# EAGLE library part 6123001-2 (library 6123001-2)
Board to Board & Mezzanine Connectors 0.8FH P08H.5 060 30/Sn TR SC Source: Datasheet
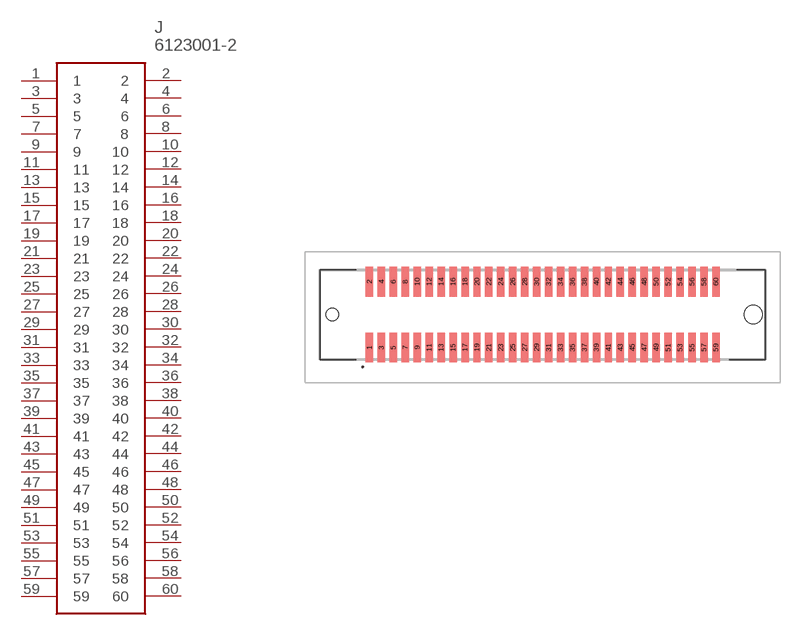
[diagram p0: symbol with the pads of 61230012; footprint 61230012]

Designator prefix J

## 6123001-2 (Arrow_Part_Number: 6123001-2; Arrow_Price-Stock: https://www.arrow.com/en/products/6123001-2/te-connectivity; Description: Board to Board & Mezzanine Connectors 0.8FH P08H.5 060 30/Sn TR SC; Height: 7.8mm; Manufacturer_Name: TE Connectivity; Manufacturer_Part_Number: 6123001-2; Mouser_Part_Number: 571-6123001-2; Mouser_Price-Stock: https://www.mouser.com/Search/Refine.aspx?Keyword=571-6123001-2)  [61230012]
1  1
2  2
3  3
4  4
5  5
6  6
7  7
8  8
9  9
10  10
11  11
12  12
13  13
14  14
15  15
16  16
17  17
18  18
19  19
20  20
21  21
22  22
23  23
24  24
25  25
26  26
27  27
28  28
29  29
30  30
31  31
32  32
33  33
34  34
35  35
36  36
37  37
38  38
39  39
40  40
41  41
42  42
43  43
44  44
45  45
46  46
47  47
48  48
49  49
50  50
51  51
52  52
53  53
54  54
55  55
56  56
57  57
58  58
59  59
60  60

## Footprint 61230012 (pad centres in mm)
6123001-2-2
smd 0.5 x 2: 1 -11.6,-2.2; 2 -11.6,2.2; 3 -10.8,-2.2; 4 -10.8,2.2; 5 -10,-2.2; 6 -10,2.2; 7 -9.2,-2.2; 8 -9.2,2.2; 9 -8.4,-2.2; 10 -8.4,2.2; 11 -7.6,-2.2; 12 -7.6,2.2; 13 -6.8,-2.2; 14 -6.8,2.2; 15 -6,-2.2; 16 -6,2.2; 17 -5.2,-2.2; 18 -5.2,2.2; 19 -4.4,-2.2; 20 -4.4,2.2; 21 -3.6,-2.2; 22 -3.6,2.2; 23 -2.8,-2.2; 24 -2.8,2.2; 25 -2,-2.2; 26 -2,2.2; 27 -1.2,-2.2; 28 -1.2,2.2; 29 -0.4,-2.2; 30 -0.4,2.2; 31 0.4,-2.2; 32 0.4,2.2; 33 1.2,-2.2; 34 1.2,2.2; 35 2,-2.2; 36 2,2.2; 37 2.8,-2.2; 38 2.8,2.2; 39 3.6,-2.2; 40 3.6,2.2; 41 4.4,-2.2; 42 4.4,2.2; 43 5.2,-2.2; 44 5.2,2.2; 45 6,-2.2; 46 6,2.2; 47 6.8,-2.2; 48 6.8,2.2; 49 7.6,-2.2; 50 7.6,2.2; 51 8.4,-2.2; 52 8.4,2.2; 53 9.2,-2.2; 54 9.2,2.2; 55 10,-2.2; 56 10,2.2; 57 10.8,-2.2; 58 10.8,2.2; 59 11.6,-2.2; 60 11.6,2.2
hole 0.83 at -14.1,0
hole 1.23 at 14.1,0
